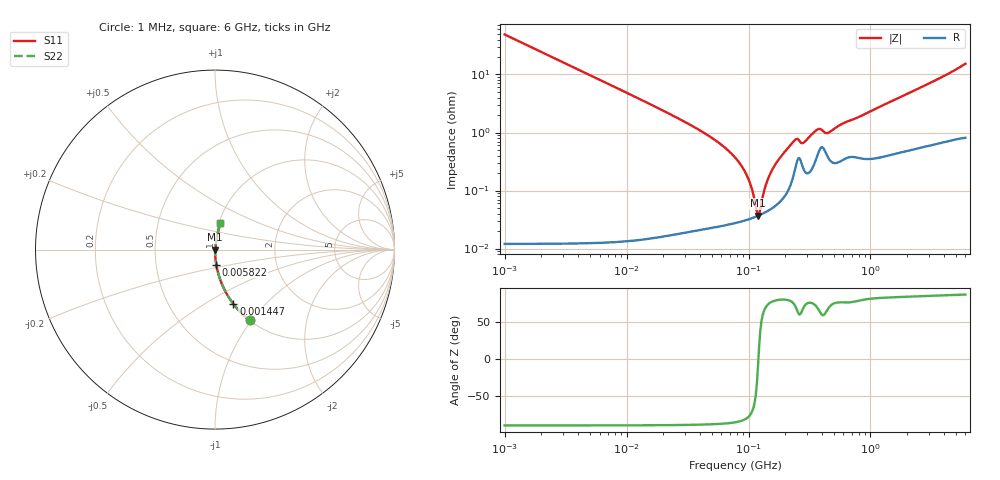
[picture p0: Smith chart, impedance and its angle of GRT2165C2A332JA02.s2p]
!Murata Part Number: GRT2165C2A332JA02
!These Parameters are Measured in Series Mode Connection
!Data Generated on Jun 19, 2026
!  o--ll--o
!Port1  Port2
!  o------o
!Operation Temp=25[degC], DC Bias Voltage=0[V]
!Freq. Start=1000[kHz] Stop=6[GHz] 401[Steps]
# Hz S RI R 50
!Freq.(Hz) S11(Real) S11(Imag) S21(Real) S21(Imag) S12(Real) S12(Imag) S22(Real) S22(Imag)
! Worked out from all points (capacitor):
!   401 points, 1 MHz to 6 GHz, reference 50 ohm
!   read as one part in series: C = 3.25 nF near 1.044 MHz
!   lowest |Z| = 37.2 mohm at 119.7 MHz (marker M1)
!   series resonance near 120.5 MHz, so ESL is about 540 pH
!   S11 on the Smith chart (normalised r, x): 1 MHz: 1.00, -0.98; 1.447 MHz: 1.00, -0.68; 5.822 MHz: 1.00, -0.17; 6 GHz: 1.02, +0.31
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1000000  0.1933 -0.3947  0.8067 0.3947  0.8067 0.3947  0.1933 -0.3947
1447343  0.1027 -0.3033  0.8973 0.3033  0.8973 0.3033  0.1027 -0.3033
4293785  0.0129 -0.1123  0.9871 0.1123  0.9871 0.1123  0.0129 -0.1123
5822046  0.0071 -0.0832  0.9929 0.0832  0.9929 0.0832  0.0071 -0.0832
1.843659e7  0.000826 -0.0259  0.9992 0.0259  0.9992 0.0259  0.000826 -0.0259
4.697123e7  0.0003 -0.00882  0.9997 0.00882  0.9997 0.00882  0.0003 -0.00882
7.745967e7  0.000288 -0.00372  0.9997 0.00372  0.9997 0.00372  0.000288 -0.00372
9.83954e7  0.000318 -0.00167  0.9997 0.00167  0.9997 0.00167  0.000318 -0.00167
1.050294e8  0.000332 -0.00113  0.9997 0.00113  0.9997 0.00113  0.000332 -0.00113
1.170949e8  0.00036 -0.000236  0.9996 0.000236  0.9996 0.000236  0.00036 -0.000236
1.196694e8  0.000367 -5.65e-05  0.9996 5.65e-05  0.9996 5.65e-05  0.000367 -5.65e-05
1.249896e8  0.000382 0.000303  0.9996 -0.000303  0.9996 -0.000303  0.000382 0.000303
1.363501e8  0.000419 0.00103  0.9996 -0.00103  0.9996 -0.00103  0.000419 0.00103
1.455431e8  0.000454 0.00159  0.9995 -0.00159  0.9995 -0.00159  0.000454 0.00159
1.732027e8  0.000596 0.00317  0.9994 -0.00317  0.9994 -0.00317  0.000596 0.00317
2.400133e8  0.00232 0.00704  0.9977 -0.00704  0.9977 -0.00704  0.00232 0.00704
2.794814e8  0.00251 0.00606  0.9975 -0.00606  0.9975 -0.00606  0.00251 0.00606
3.325952e8  0.00247 0.00909  0.9975 -0.00909  0.9975 -0.00909  0.00247 0.00909
3.789555e8  0.00491 0.0104  0.9951 -0.0104  0.9951 -0.0104  0.00491 0.0104
4.509737e8  0.00373 0.00914  0.9963 -0.00914  0.9963 -0.00914  0.00373 0.00914
1.428092e9  0.00511 0.0328  0.9949 -0.0328  0.9949 -0.0328  0.00511 0.0328
6e9  0.0304 0.1474  0.9696 -0.1474  0.9696 -0.1474  0.0304 0.1474
